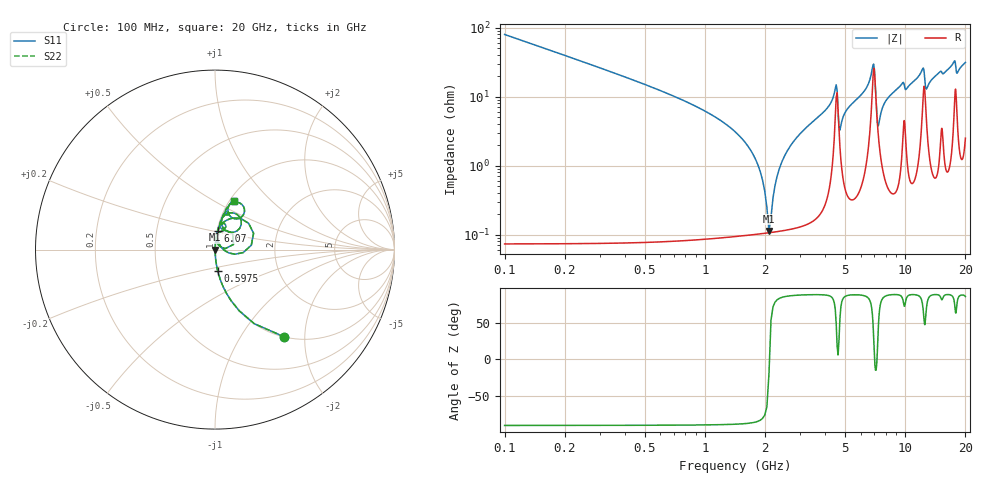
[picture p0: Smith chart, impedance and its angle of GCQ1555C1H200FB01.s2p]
!Murata Part Number: GCQ1555C1H200FB01
!These Parameters are Measured in Series Mode Connection
!Data Generated on Jan 08, 2026
!  o--ll--o
!Port1  Port2
!  o------o
!Operation Temp=25[degC], DC Bias Voltage=0[V]
!Freq. Start=100[MHz] Stop=20[GHz] 401[Steps]
# Hz S RI R 50
!Freq.(Hz) S11(Real) S11(Imag) S21(Real) S21(Imag) S12(Real) S12(Imag) S22(Real) S22(Imag)
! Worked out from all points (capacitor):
!   401 points, 100 MHz to 20 GHz, reference 50 ohm
!   read as one part in series: C = 20 pF near 199.5 MHz
!   lowest |Z| = 113 mohm at 2.09 GHz (marker M1)
!   series resonance near 2.1 GHz, so ESL is about 290 pH
!   S11 on the Smith chart (normalised r, x): 100 MHz: 1.00, -1.59; 597.5 MHz: 1.00, -0.25; 6.07 GHz: 1.01, +0.22; 20 GHz: 1.05, +0.62
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1e8  0.3868 -0.4865  0.6132 0.4865  0.6132 0.4865  0.3868 -0.4865
5.975e8  0.0155 -0.1205  0.9845 0.1205  0.9845 0.1205  0.0155 -0.1205
1.64225e9  0.00134 -0.019  0.9987 0.019  0.9987 0.019  0.00134 -0.019
1.84125e9  0.00112 -0.0101  0.9989 0.0101  0.9989 0.0101  0.00112 -0.0101
2.09e9  0.00106 -0.000379  0.9989 0.000379  0.9989 0.000379  0.00106 -0.000379
2.53775e9  0.00138 0.0149  0.9986 -0.0149  0.9986 -0.0149  0.00138 0.0149
3.43325e9  0.00332 0.0422  0.9967 -0.0422  0.9967 -0.0422  0.00332 0.0422
4.478e9  0.0582 0.1084  0.9418 -0.1084  0.9418 -0.1084  0.0582 0.1084
4.7765e9  0.0134 0.0349  0.9866 -0.0349  0.9866 -0.0349  0.0134 0.0349
6.07e9  0.0165 0.1057  0.9835 -0.1057  0.9835 -0.1057  0.0165 0.1057
6.7665e9  0.0865 0.1729  0.9135 -0.1729  0.9135 -0.1729  0.0865 0.1729
6.9655e9  0.215 0.0908  0.785 -0.0908  0.785 -0.0908  0.215 0.0908
7.3635e9  0.0257 0.0271  0.9743 -0.0271  0.9743 -0.0271  0.0257 0.0271
8.259e9  0.0138 0.0957  0.9862 -0.0957  0.9862 -0.0957  0.0138 0.0957
1.005e10  0.0393 0.1156  0.9607 -0.1156  0.9607 -0.1156  0.0393 0.1156
1.2239e10  0.1132 0.2009  0.8868 -0.2009  0.8868 -0.2009  0.1132 0.2009
1.27365e10  0.0624 0.104  0.9376 -0.104  0.9376 -0.104  0.0624 0.104
1.338325e10  0.0364 0.1587  0.9636 -0.1587  0.9636 -0.1587  0.0364 0.1587
1.67165e10  0.0725 0.2412  0.9275 -0.2412  0.9275 -0.2412  0.0725 0.2412
1.7612e10  0.1418 0.2574  0.8582 -0.2574  0.8582 -0.2574  0.1418 0.2574
1.815925e10  0.0884 0.1826  0.9116 -0.1826  0.9116 -0.1826  0.0884 0.1826
2e10  0.1066 0.2712  0.8934 -0.2712  0.8934 -0.2712  0.1066 0.2712
